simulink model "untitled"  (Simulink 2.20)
settings: Solver=ode45  StartTime=0.0  StopTime=10.0  RelTol=1e-3  AbsTol=1e-6

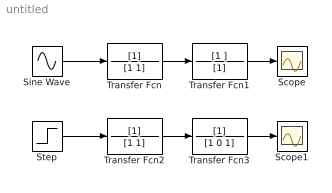
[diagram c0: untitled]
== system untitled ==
  Scope : Scope
  Scope1 : Scope
  Sine Wave : Sin  Amplitude=1  Frequency=1  Phase=0  SampleTime=0
  Step : Step  Time=0  Before=0  After=1
  Transfer Fcn : TransferFcn  Numerator=[1]  Denominator=[1 1]
  Transfer Fcn1 : TransferFcn  Numerator=[1 ]  Denominator=[1]
  Transfer Fcn2 : TransferFcn  Numerator=[1]  Denominator=[1 1]
  Transfer Fcn3 : TransferFcn  Numerator=[1]  Denominator=[1 0 1]
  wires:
  Sine Wave/1 -> Transfer Fcn/1
  Transfer Fcn/1 -> Transfer Fcn1/1
  Transfer Fcn1/1 -> Scope/1
  Step/1 -> Transfer Fcn2/1
  Transfer Fcn2/1 -> Transfer Fcn3/1
  Transfer Fcn3/1 -> Scope1/1
